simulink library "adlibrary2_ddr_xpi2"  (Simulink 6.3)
undefined symbols (not defined in the file or in its folder): adlibrary2, ADM, blackbox2, blue, DDR, ddr64xpi_config, eb5a5517, gcbh, II, Inactive, memsize, SDRAM, Simulation, Subsystem, VER_STRING_GOES_HERE, white, xlBlockLoadCallback, XRC, XRM
libraries: xbsIndex_r4 x28, adlibrary2_ddr_xpi0 x1

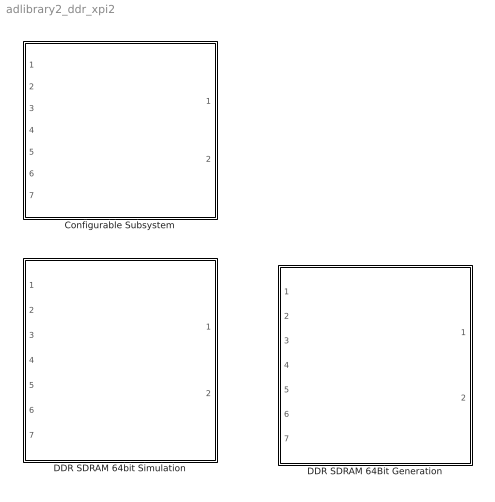
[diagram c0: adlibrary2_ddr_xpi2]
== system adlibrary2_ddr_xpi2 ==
  Configurable Subsystem : Subsystem  Tag=configX  BlockChoice=DDR SDRAM 64bit Simulation  mask{memsize=memsize}
      mask prompts: memsize "Simulation Ram Size (Mb)"
  DDR SDRAM 64Bit Generation : Subsystem
  DDR SDRAM 64bit Simulation : Subsystem  mask{memsize=memsize}
      mask prompts: memsize "Simulation Ram Size (Mb)"

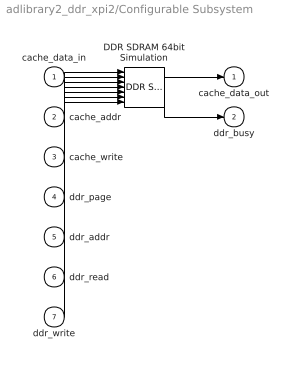
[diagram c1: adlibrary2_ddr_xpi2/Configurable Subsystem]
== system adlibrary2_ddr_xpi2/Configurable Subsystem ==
  cache_data_in : Inport
  cache_addr : Inport  Port=2
  cache_write : Inport  Port=3
  ddr_page : Inport  Port=4
  ddr_addr : Inport  Port=5
  ddr_read : Inport  Port=6
  ddr_write : Inport  Port=7
  DDR SDRAM 64bit Simulation : adlibrary2_ddr_xpi0/DDR SDRAM 64bit Simulation  memsize=memsize
  cache_data_out : Outport
  ddr_busy : Outport  Port=2
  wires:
  cache_data_in/1 -> DDR SDRAM 64bit Simulation/1
  cache_addr/1 -> DDR SDRAM 64bit Simulation/2
  cache_write/1 -> DDR SDRAM 64bit Simulation/3
  ddr_page/1 -> DDR SDRAM 64bit Simulation/4
  ddr_addr/1 -> DDR SDRAM 64bit Simulation/5
  ddr_read/1 -> DDR SDRAM 64bit Simulation/6
  ddr_write/1 -> DDR SDRAM 64bit Simulation/7
  DDR SDRAM 64bit Simulation/1 -> cache_data_out/1
  DDR SDRAM 64bit Simulation/2 -> ddr_busy/1

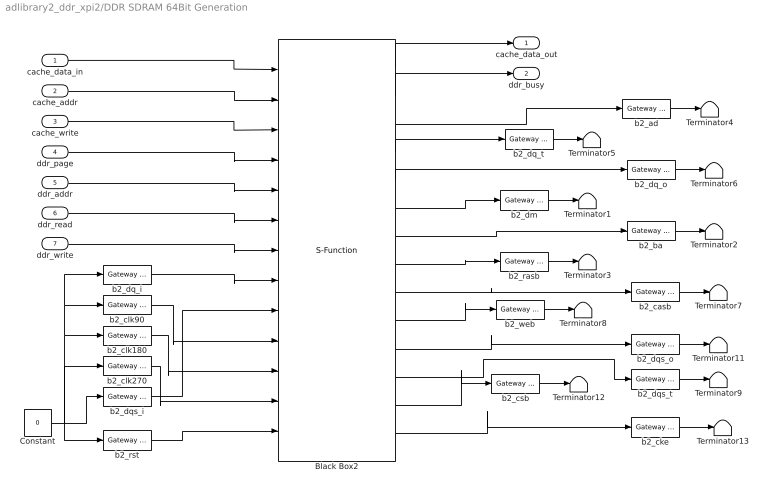
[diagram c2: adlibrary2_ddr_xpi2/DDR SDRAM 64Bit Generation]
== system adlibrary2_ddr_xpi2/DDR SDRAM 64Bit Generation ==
  cache_data_in : Inport
  cache_addr : Inport  Port=2
  cache_write : Inport  Port=3
  ddr_page : Inport  Port=4
  ddr_addr : Inport  Port=5
  ddr_read : Inport  Port=6
  ddr_write : Inport  Port=7
  Black Box2 : S-Function  LoadFcn=xlBlockLoadCallback(gcbh);  FunctionName=sysgen  Parameters=ptable_  mask(Xilinx Black Box Block){infoedit=Incorporates black box HDL and simulation model into a System Generator design.<P><P>You must supply a Black Box with certain information about the HDL component you would like to bring into System Generator. This information is provided through a Matlab function.<P><P>When "Simulation mode" is set to "Inactive", you will typically want to provide a separate simulation model by using a Simulation 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, init_code=ddr64xpi_config, sim_method=Inactive, sim_method_sgadvanced=, engine_block=, xl_use_area=off, xl_use_area_sgadvanced=, xl_area=[0,0,0,0,0,0,0], block_version=VER_STRING_GOES_HERE, has_advanced_control=0, sggui_pos=20,20,356,367, block_type=blackbox2, sg_icon_stat=135,483,13,14,white,blue,0,eb5a5517, sg_mask_display=fprintf('','COMMENT: begin icon graphics '); patch([0 135 135 0 ],[0 0 483 483 ],[0.77 0.82 0.91]); patch([31 9 41 9 31 67 77 87 125 95 66 45 77 45 66 95 125 87 77 67 31 ],[189 211 243 275 297 297 287 297 297 267 296 275 243 211 190 219 189 189 199 189 189 ],[0.98 0.96 0.92]); plot([0 0 135 135 0 ],[0 483 483 0 0 ]); fprintf('','COMMENT: end icon graphics');  fprintf('','COMMENT: begin icon text '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, sg_list_contents=, adlocb_devid=4, ddr_size=64}
      mask prompts: infoedit ""; init_code "Block configuration m-function"; sim_method "Simulation mode"; engine_block "HDL co-simulator to use  (specify helper block by name)"; xl_use_area "Define FPGA area for resource estimation"; xl_area "FPGA area [slices, FFs, BRAMs, LUTs, IOBs, emb. mults, TBUFs]"; block_version ""; has_advanced_control ""; sggui_pos ""; block_type ""; sg_icon_stat ""; sg_mask_display ""; sg_list_contents ""; adlocb_devid "ADLOCB DEV ID"; ddr_size "DDR BANK SIZE"
      mask help: Incorporates black box HDL and simulation model into a System Generator design. You must supply a Black Box with certain information about the HDL component you would like to bring into System Generator. This information is provided through a Matlab function. When "Simulation mode" is set to "Inactive", you will typically want to provide a separate simulation model by using a Simulation Multiplexer. When "Simulation mode" is set to "External co-simulator", you must include a ModelSim block in the design.
      mask init:
      | xlMungeMaskParams;
      | 
      | mdlPath = xlGetMdlDir(bdroot);
      | 
      | refBlk = get_param(gcb,'referenceBlock');
      | if (isempty(refBlk) | strncmp(refBlk,'xbsIndex',8))
      | srcPath = mdlPath;
      | else
      | srcPath = xlPathToReference;
      | if (isempty(srcPath))
      | srcPath = mdlPath;
      | end
      | end
      | 
      | if (sim_method==3)
      | validEngineBlock = 0;
      | try
      | engineBlock = xlBlockNameRelPath(get_param(gcb,'Parent'),engine_block);
      | catch
      | engineBlock = '//';
      | end
      | try 
      | engineWorkDir = get_param(engineBlock,'dir');
      | validEngineBlock = 1;
      | engine_handle = get_param(engineBlock,'Handle');
      | catch
      | end
      | end
      | 
      | % build black box config function
      | block_config = ['sysgen:black_box_config:' init_code];
      | 
      | serialized_declarations = '{''engine_handle''=>''Double'',''sim_method''=>''Int'',''validEngineBlock''=>''Int'',''engineWorkDir''=>''String'',''engine_block''=>''String'',''init_code''=>''String'',''mdlPath''=>''String'',''srcPath''=>''String'',''block_config''=>''String'',}';
      | ptable_ = xlblockprep(get_param(gcb, 'MaskWSVariables'));
  Constant : Constant  Value=0
  Terminator{1..9,11..13} (12 alike) : Terminator
  b2_ad : xbsIndex_r4/Gateway Out  hdl_port=on  timing_constraint=None  locs_specified=off  LOCs={}  block_type=gatewayout
  b2_ba : xbsIndex_r4/Gateway Out  hdl_port=on  timing_constraint=None  locs_specified=off  LOCs={}  block_type=gatewayout
  b2_casb : xbsIndex_r4/Gateway Out  hdl_port=on  timing_constraint=None  locs_specified=off  LOCs={}  block_type=gatewayout
  b2_cke : xbsIndex_r4/Gateway Out  hdl_port=on  timing_constraint=None  locs_specified=off  LOCs={}  block_type=gatewayout
  b2_clk180 : xbsIndex_r4/Gateway In  arith_type=Boolean  n_bits=64  bin_pt=0  period=ad_get_simulink_period  dbl_ovrd=off  timing_constraint=None  locs_specified=off  LOCs={}  block_type=gatewayin
  b2_clk270 : xbsIndex_r4/Gateway In  arith_type=Boolean  n_bits=64  bin_pt=0  period=ad_get_simulink_period  dbl_ovrd=off  timing_constraint=None  locs_specified=off  LOCs={}  block_type=gatewayin
  b2_clk90 : xbsIndex_r4/Gateway In  arith_type=Boolean  n_bits=64  bin_pt=0  period=ad_get_simulink_period  dbl_ovrd=off  timing_constraint=None  locs_specified=off  LOCs={}  block_type=gatewayin
  b2_csb : xbsIndex_r4/Gateway Out  hdl_port=on  timing_constraint=None  locs_specified=off  LOCs={}  block_type=gatewayout
  b2_dm : xbsIndex_r4/Gateway Out  hdl_port=on  timing_constraint=None  locs_specified=off  LOCs={}  block_type=gatewayout
  b2_dq_i : xbsIndex_r4/Gateway In  arith_type=Unsigned  n_bits=64  bin_pt=0  period=ad_get_simulink_period  dbl_ovrd=off  timing_constraint=None  locs_specified=off  LOCs={}  block_type=gatewayin
  b2_dq_o : xbsIndex_r4/Gateway Out  hdl_port=on  timing_constraint=None  locs_specified=off  LOCs={}  block_type=gatewayout
  b2_dq_t : xbsIndex_r4/Gateway Out  hdl_port=on  timing_constraint=None  locs_specified=off  LOCs={}  block_type=gatewayout
  b2_dqs_i : xbsIndex_r4/Gateway In  arith_type=Unsigned  n_bits=8  bin_pt=0  period=ad_get_simulink_period  dbl_ovrd=off  timing_constraint=None  locs_specified=off  LOCs={}  block_type=gatewayin
  b2_dqs_o : xbsIndex_r4/Gateway Out  hdl_port=on  timing_constraint=None  locs_specified=off  LOCs={}  block_type=gatewayout
  b2_dqs_t : xbsIndex_r4/Gateway Out  hdl_port=on  timing_constraint=None  locs_specified=off  LOCs={}  block_type=gatewayout
  b2_rasb : xbsIndex_r4/Gateway Out  hdl_port=on  timing_constraint=None  locs_specified=off  LOCs={}  block_type=gatewayout
  b2_rst : xbsIndex_r4/Gateway In  arith_type=Boolean  n_bits=64  bin_pt=0  period=ad_get_simulink_period  dbl_ovrd=off  timing_constraint=None  locs_specified=off  LOCs={}  block_type=gatewayin
  b2_web : xbsIndex_r4/Gateway Out  hdl_port=on  timing_constraint=None  locs_specified=off  LOCs={}  block_type=gatewayout
  cache_data_out : Outport
  ddr_busy : Outport  Port=2
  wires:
  b2_cke/1 -> Terminator13/1
  b2_csb/1 -> Terminator12/1
  b2_dqs_o/1 -> Terminator11/1
  b2_web/1 -> Terminator8/1
  b2_casb/1 -> Terminator7/1
  b2_rasb/1 -> Terminator3/1
  b2_ba/1 -> Terminator2/1
  b2_dm/1 -> Terminator1/1
  b2_dq_o/1 -> Terminator6/1
  b2_dq_t/1 -> Terminator5/1
  b2_ad/1 -> Terminator4/1
  Black Box2/2 -> ddr_busy/1
  Black Box2/1 -> cache_data_out/1
  ddr_write/1 -> Black Box2/7
  ddr_read/1 -> Black Box2/6
  ddr_addr/1 -> Black Box2/5
  ddr_page/1 -> Black Box2/4
  cache_write/1 -> Black Box2/3
  cache_addr/1 -> Black Box2/2
  cache_data_in/1 -> Black Box2/1
  b2_dq_i/1 -> Black Box2/8
  Constant/1 -> b2_dq_i/1, b2_clk90/1, b2_clk180/1, b2_clk270/1, b2_dqs_i/1, b2_rst/1
  b2_dqs_t/1 -> Terminator9/1
  Black Box2/3 -> b2_ad/1
  Black Box2/4 -> b2_dq_t/1
  Black Box2/5 -> b2_dq_o/1
  Black Box2/6 -> b2_dm/1
  Black Box2/7 -> b2_ba/1
  Black Box2/8 -> b2_rasb/1
  Black Box2/9 -> b2_casb/1
  Black Box2/10 -> b2_web/1
  Black Box2/11 -> b2_dqs_o/1
  Black Box2/12 -> b2_dqs_t/1
  Black Box2/13 -> b2_csb/1
  Black Box2/14 -> b2_cke/1
  b2_dqs_i/1 -> Black Box2/9
  b2_clk90/1 -> Black Box2/10
  b2_clk180/1 -> Black Box2/11
  b2_clk270/1 -> Black Box2/12
  b2_rst/1 -> Black Box2/13

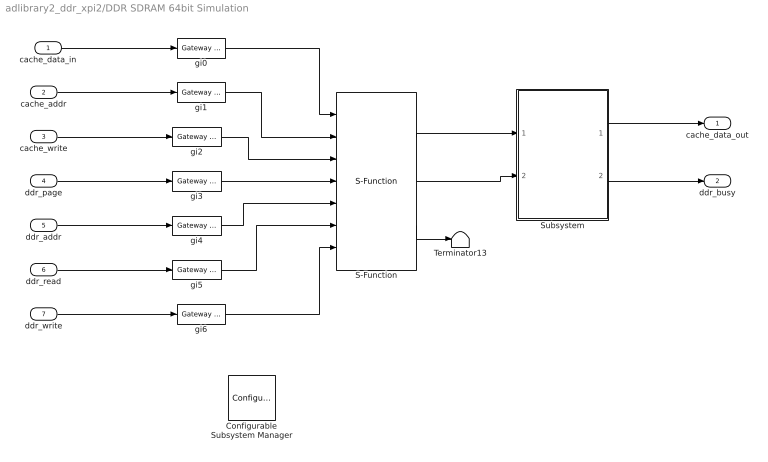
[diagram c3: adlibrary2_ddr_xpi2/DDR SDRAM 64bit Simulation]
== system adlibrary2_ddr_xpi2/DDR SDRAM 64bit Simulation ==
  cache_data_in : Inport
  cache_addr : Inport  Port=2
  cache_write : Inport  Port=3
  ddr_page : Inport  Port=4
  ddr_addr : Inport  Port=5
  ddr_read : Inport  Port=6
  ddr_write : Inport  Port=7
  Configurable Subsystem Manager : xbsIndex_r4/Configurable Subsystem Manager  Tag=xcfgMgr  block_type=configsubsys
  S-Function : S-Function  FunctionName=ddr64  Parameters=memsize,0
  Subsystem : Subsystem  AncestorBlock=adlibrary2/ADM-XRC-II/XRM DDR SDRAM /DDR SDRAM 64bit Simulation/Subsystem
  Terminator13 : Terminator
  gi{0..6} (7 alike) : xbsIndex_r4/Gateway Out  hdl_port=off  timing_constraint=None  locs_specified=off  LOCs={}  block_type=gatewayout
  cache_data_out : Outport
  ddr_busy : Outport  Port=2
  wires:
  cache_data_in/1 -> gi0/1
  cache_addr/1 -> gi1/1
  cache_write/1 -> gi2/1
  ddr_page/1 -> gi3/1
  ddr_addr/1 -> gi4/1
  ddr_read/1 -> gi5/1
  ddr_write/1 -> gi6/1
  gi0/1 -> S-Function/1
  gi1/1 -> S-Function/2
  gi2/1 -> S-Function/3
  gi3/1 -> S-Function/4
  gi4/1 -> S-Function/5
  gi5/1 -> S-Function/6
  gi6/1 -> S-Function/7
  S-Function/2 -> Subsystem/2(In2)
  S-Function/1 -> Subsystem/1(In1)
  Subsystem/1(Out1) -> cache_data_out/1
  Subsystem/2(Out2) -> ddr_busy/1
  S-Function/3 -> Terminator13/1

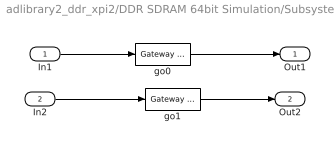
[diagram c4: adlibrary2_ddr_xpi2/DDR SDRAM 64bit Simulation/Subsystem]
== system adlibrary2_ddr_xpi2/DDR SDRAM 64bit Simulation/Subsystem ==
  In1 : Inport
  In2 : Inport  Port=2
  go0 : xbsIndex_r4/Gateway In  arith_type=Unsigned  n_bits=32  bin_pt=0  period=ad_get_simulink_period  dbl_ovrd=off  timing_constraint=None  locs_specified=off  LOCs={}  block_type=gatewayin
  go1 : xbsIndex_r4/Gateway In  arith_type=Boolean  n_bits=32  bin_pt=0  period=ad_get_simulink_period  dbl_ovrd=off  timing_constraint=None  locs_specified=off  LOCs={}  block_type=gatewayin
  Out1 : Outport
  Out2 : Outport  Port=2
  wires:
  go1/1 -> Out2/1
  go0/1 -> Out1/1
  In2/1 -> go1/1
  In1/1 -> go0/1
